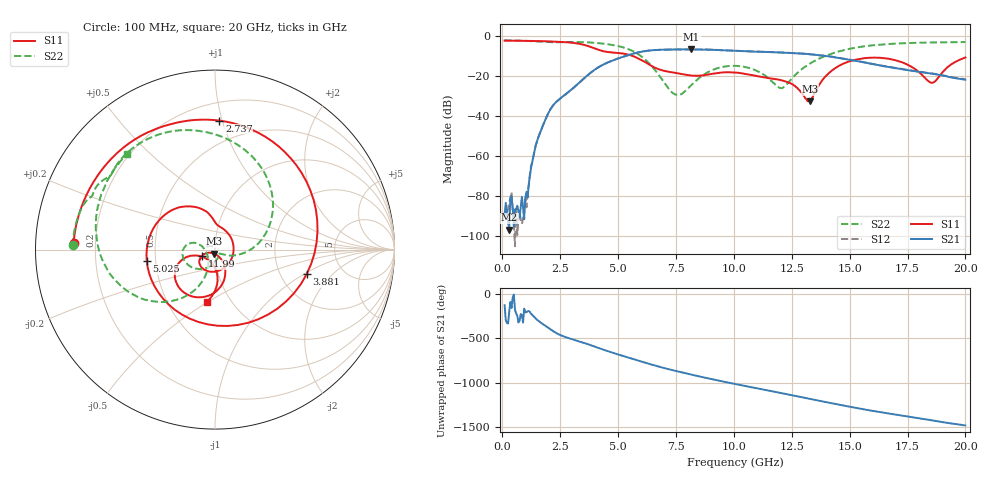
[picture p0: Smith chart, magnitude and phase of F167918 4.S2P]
!  2-Port S-parameters saved by WinCal
! VAR MeasName=S-Parameters (CALIBRATED_DATA) read from VNA (N5242A)
! VAR MeasDate=2016-11-22 10:25:03
! VAR NAME=F167918 4
! VAR FILENAME=F167918 4.S2P
! VAR DATE=2016-11-22 10:25:03
! VAR PHYS_PORTS=1,2
# Hz S DB R 50
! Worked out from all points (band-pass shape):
!   401 points, 100 MHz to 20 GHz, reference 50 ohm
!   highest |S21| = -6.46 dB at 8.159 GHz (marker M1); lowest = -96.9 dB at 299 MHz (marker M2)
!   |S21| within 3 dB of the highest: 5.411 GHz to 13.73 GHz (8.32 GHz wide, 86.9 % of centre)
!   lowest |S11| = -32.5 dB at 13.28 GHz (marker M3), VSWR 1.05, Z = 49.6 - j2.33 ohm
!   |S11| at or under -10 dB: 5.678 GHz to end of sweep
!   |S22| runs from -29.3 to -2.0 dB; largest |S21 - S12| = 0.0041
!   S11 on the Smith chart (normalised r, x): 100 MHz: 0.12, +0.02; 2.737 GHz: 0.33, +0.98; 3.881 GHz: 2.80, -1.06; 5.025 GHz: 0.45, -0.07; 11.99 GHz: 0.86, -0.07; 20 GHz: 0.77, -0.50
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1e8  -2.07 177.3  -89.77 -130.8  -88.20 48.1  -2.00 178.3
2.99e8  -2.09 172.0  -96.94 156.0  -83.32 -129.0  -2.02 174.9
9.955e8  -2.20 153.2  -80.93 149.3  -81.50 -169.7  -2.17 162.9
1.692e9  -2.34 132.0  -46.42 26.7  -46.43 26.6  -2.52 152.3
2.73675e9  -2.86 88.0  -29.03 -129.4  -29.04 -129.7  -2.78 136.9
3.43325e9  -3.94 36.7  -22.01 174.0  -22.02 173.9  -2.83 121.5
3.881e9  -5.53 -14.9  -17.61 135.1  -17.60 135.1  -3.08 109.7
4.3785e9  -7.44 -88.1  -14.00 89.1  -13.95 89.0  -3.64 94.7
5.02525e9  -8.28 -170.7  -10.95 34.4  -10.92 33.9  -4.89 70.9
5.871e9  -11.01 121.1  -7.99 -32.6  -8.01 -32.9  -8.91 28.7
6.7665e9  -16.48 89.1  -6.69 -100.5  -6.72 -100.7  -19.44 -18.1
7.463e9  -18.23 65.3  -6.53 -146.7  -6.54 -146.8  -29.05 -38.7
8.1595e9  -19.59 12.5  -6.46 170.6  -6.48 170.6  -24.49 -81.7
9.10475e9  -18.67 -72.2  -6.70 116.1  -6.68 116.0  -16.66 -133.0
1.005e10  -18.06 -124.5  -7.16 65.0  -7.15 65.1  -14.74 -170.5
1.199025e10  -21.80 -152.3  -8.02 -34.0  -7.99 -34.1  -25.86 -163.1
1.328375e10  -32.52 -97.5  -8.90 -101.9  -8.90 -101.7  -13.61 -113.1
1.338325e10  -30.85 -77.0  -9.00 -107.3  -9.01 -107.0  -12.93 -114.4
1.4627e10  -14.18 -77.8  -10.93 -171.8  -10.88 -171.6  -7.21 -138.3
1.67165e10  -11.29 -144.6  -15.33 92.9  -15.31 92.9  -3.77 179.6
1.855725e10  -23.26 -124.5  -18.62 16.9  -18.57 17.0  -3.02 151.4
2e10  -10.53 -99.0  -21.67 -40.4  -21.48 -40.3  -2.82 132.6
